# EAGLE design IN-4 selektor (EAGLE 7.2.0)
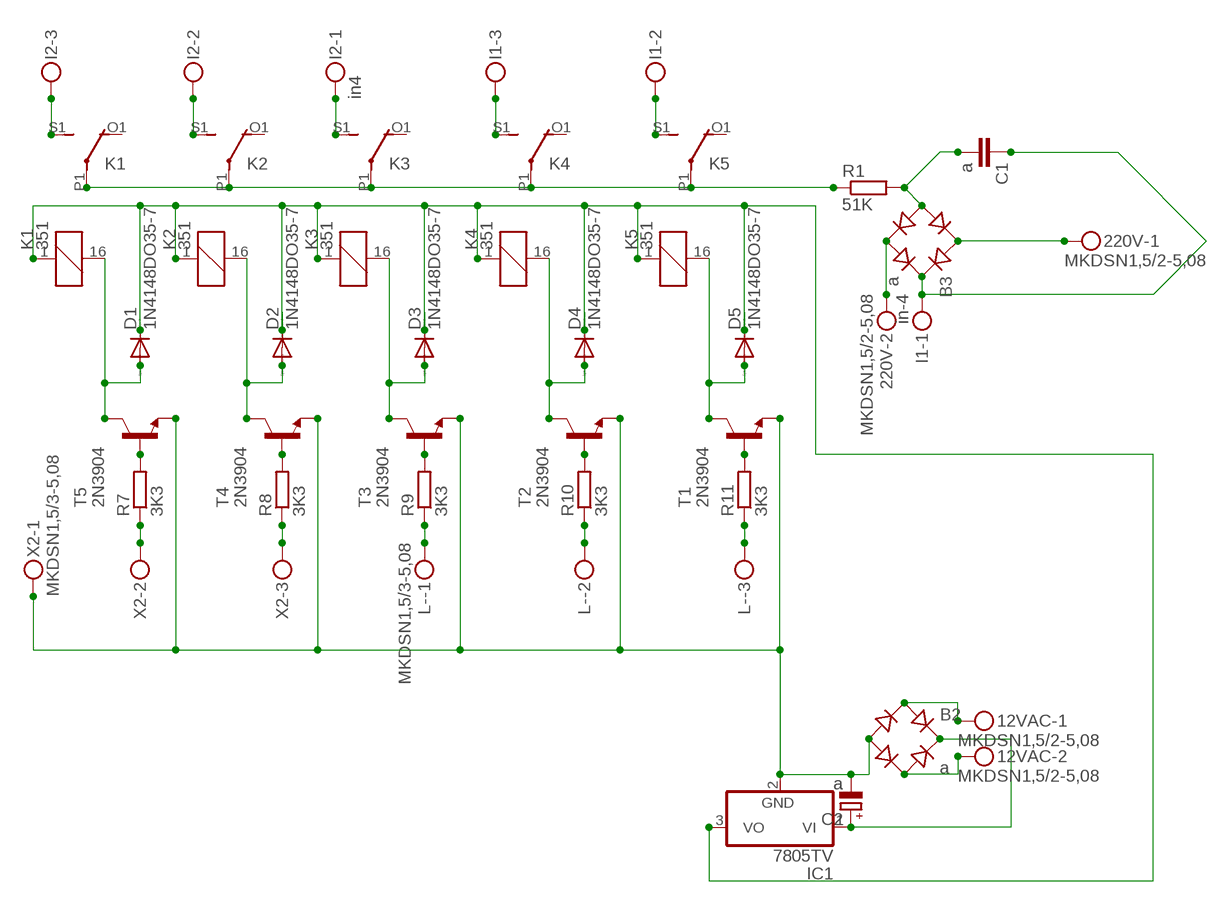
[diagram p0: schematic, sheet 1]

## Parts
12VAC  MKDSN1,5/2-5,08  [MKDSN1,5/2-5,08]
220V  MKDSN1,5/2-5,08  [MKDSN1,5/2-5,08]
B2  a  RB1A  [RB1A]
B3  a  RB1A  [RB1A]
C1  a  C-EU050-030X075  [C050-030X075]
C2  a  CPOL-EUE7.5-16  [E7,5-16]
D1  1N4148DO35-7  [DO35-7]
D2  1N4148DO35-7  [DO35-7]
D3  1N4148DO35-7  [DO35-7]
D4  1N4148DO35-7  [DO35-7]
D5  1N4148DO35-7  [DO35-7]
I1  in-4  MKDSN1,5/3-5,08  [MKDSN1,5/3-5,08]
I2  in4  MKDSN1,5/3-5,08  [MKDSN1,5/3-5,08]
IC1  7805TV  [TO220V]
K1  351  [351]
K2  351  [351]
K3  351  [351]
K4  351  [351]
K5  351  [351]
L-  MKDSN1,5/3-5,08  [MKDSN1,5/3-5,08]
R1  51K  R-EU_0207/10  [0207/10]
R7  3K3  R-EU_0204/5  [0204/5]
R8  3K3  R-EU_0204/5  [0204/5]
R9  3K3  R-EU_0204/5  [0204/5]
R10  3K3  R-EU_0204/5  [0204/5]
R11  3K3  R-EU_0204/5  [0204/5]
T1  2N3904  [TO92]
T2  2N3904  [TO92]
T3  2N3904  [TO92]
T4  2N3904  [TO92]
T5  2N3904  [TO92]
X2  MKDSN1,5/3-5,08  [MKDSN1,5/3-5,08]

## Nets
N$2: R8.2 T4.2(B)
N$3: R7.2 T5.2(B)
N$4: R9.2 T3.2(B)
N$5: R10.2 T2.2(B)
N$6: R11.2 T1.2(B)
N$7: 220V.1 B3.AC1
N$8: B3.+ C1.1 I1.1
N$9: K1.P1(2:P) K2.P1(2:P) K3.P1(2:P) K4.P1(2:P) K5.P1(2:P) R1.1
N$10: I2.3 K1.S1(2:S)
N$11: I2.2 K2.S1(2:S)
N$12: I2.1 K3.S1(2:S)
N$13: I1.3 K4.S1(2:S)
N$14: I1.2 K5.S1(2:S)
N$15: 220V.2 B3.AC2
N$16: R7.1 X2.2
N$17: B3.- C1.2 R1.2
N$19: B2.- C2.- IC1.2(GND) T1.3(E) T2.3(E) T3.3(E) T4.3(E) T5.3(E) X2.1
N$20: D1.A K1.16 T5.1(C)
N$22: R8.1 X2.3
N$23: L-.1 R9.1
N$25: D2.A K2.16 T4.1(C)
N$27: 12VAC.1 B2.AC1
N$28: 12VAC.2 B2.AC2
N$29: B2.+ C2.+ IC1.1(VI)
N$30: L-.2 R10.1
N$31: L-.3 R11.1
N$32: D3.A K3.16 T3.1(C)
N$34: D4.A K4.16 T2.1(C)
N$36: D5.A K5.16 T1.1(C)
N$37: D1.C D2.C D3.C D4.C D5.C IC1.3(VO) K1.1 K2.1 K3.1 K4.1 K5.1
Unconnected: K1.O1(2:O) K1.O2(3:O) K1.P2(3:P) K1.S2(3:S) K2.O1(2:O) K2.O2(3:O) K2.P2(3:P) K2.S2(3:S) K3.O1(2:O) K3.O2(3:O) K3.P2(3:P) K3.S2(3:S) K4.O1(2:O) K4.O2(3:O) K4.P2(3:P) K4.S2(3:S) K5.O1(2:O) K5.O2(3:O) K5.P2(3:P) K5.S2(3:S)

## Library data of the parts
12VAC 220V = con-phoenix-508:MKDSN1,5/2-5,08: MKDSN 1,5/ 2-5,08 Printklemme
B2 B3 = rectifier:RB1A: RECTIFIER 1 A
C1 = rcl:C-EU: CAPACITOR, European symbol
C2 = resistor:CPOL-EU: POLARIZED CAPACITOR, European symbol
D1-D5 = diode:1N4148: DIODE
I1 I2 L- X2 = con-phoenix-508:MKDSN1,5/3-5,08: MKDSN 1,5/ 3-5,08 Printklemme Nennstrom: 13,5 A Nennspannung: 250 V Rastermaß: 5,08 mm Polzahl: 3 Anschlussart: Schraubanschluss Montage: Löten Anschlussrichtung Leiter/Platine: 0 ° Artikelnummer: 1729131 Source: http://eshop.phoenixcontact.com .. 1729131.pdf
IC1 = linear:78*: Positive VOLTAGE REGULATOR Source: http://cache.national.com/ds/LM/LM78L05.pdf http://www.fairchildsemi.com/ds/LM/LM7805.pdf
K1-K5 = relay:351: RELAY 2 x switch, Omron; OC_FARNELL: unknown; OC_NEWARK: unknown
R1 R7-R11 = rcl:R-EU_: RESISTOR, European symbol
T1-T5 = transistor-neu-to92:2N3904: NPN TRANSISTOR

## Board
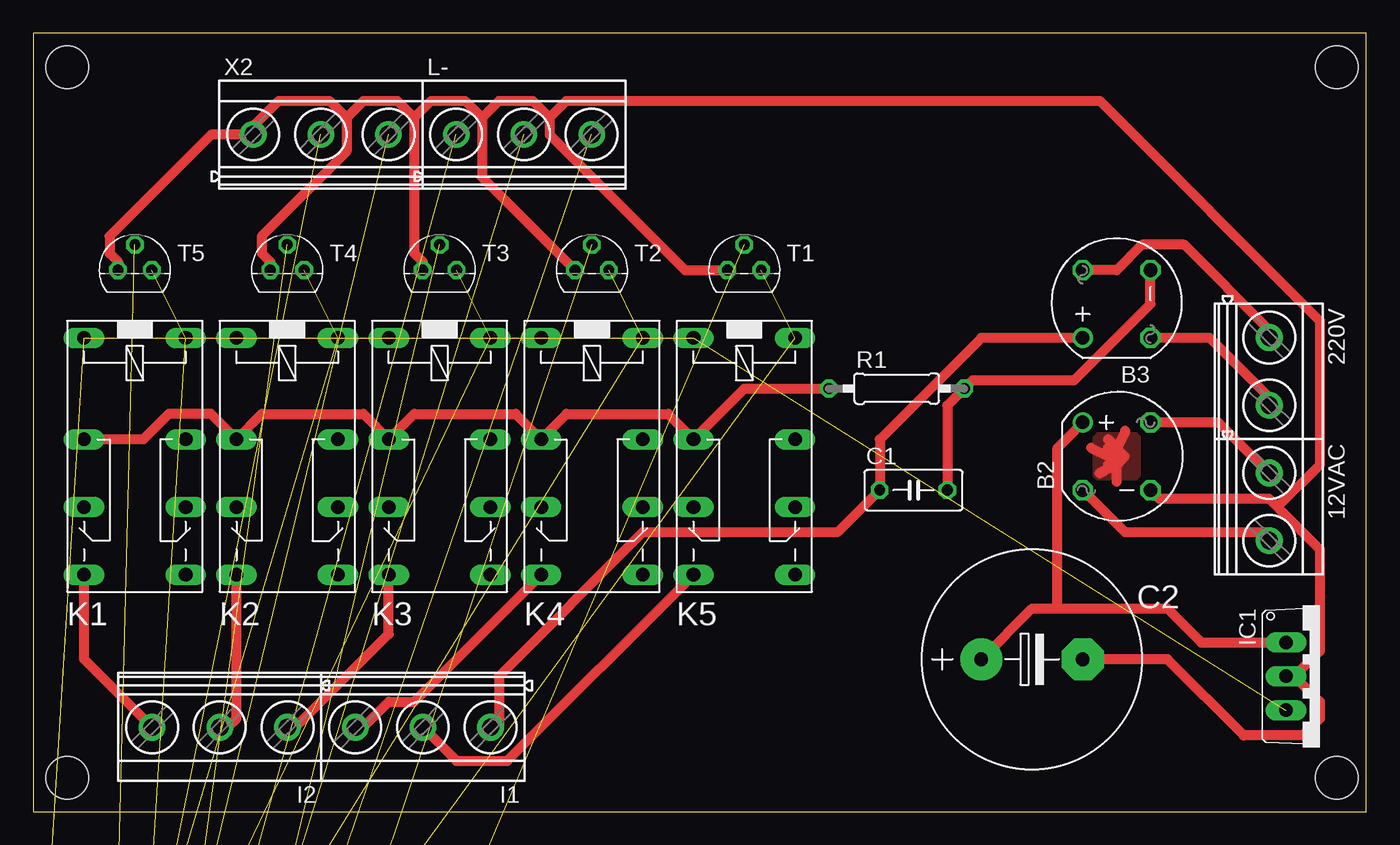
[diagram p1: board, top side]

Size 100 x 58.41 mm. Coordinates in mm from the lower left corner, seen from the top.
Outline: 0,0 100,0 100,58.41 0,58.41 0,0
Copper layers (1*16): Top 0.035mm / dielectric 1.5mm / Bottom 0.035mm
Design rules "default *": minimum track width 30mil, minimum drill 24mil, track to track 20mil, track to pad 20mil, pad to pad 20mil, via to via 20mil, smd to smd 20mil, copper to edge 50mil, drill to drill 20mil, minimum pad ring 10mil, minimum via ring 8mil, stop-mask expansion 4mil, vias tented up to drill 0mil, thermal gap 10mil
Holes 3.2 mm at 2.54,2.54 97.79,2.54 97.79,55.88 2.54,55.88

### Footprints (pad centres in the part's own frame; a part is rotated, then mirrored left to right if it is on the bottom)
MKDSN1,5/2-5,08 = drill 1.3 pad 2: 1 -2.561,0.025; 2 2.519,0.025
RB1A = drill 1.016: + -2.54,2.54 | drill 1.016 octagon: - 2.54,-2.54; AC1 2.54,2.54; AC2 -2.54,-2.54
C050-030X075 = drill 0.813 octagon: 1 -2.54,0; 2 2.54,0
E7,5-16 = drill 1.016 pad 3.15: + -3.81,0 | drill 1.016 pad 3.15 octagon: - 3.81,0
DO35-7 = drill 0.813 long: A 3.81,0; C -3.81,0
MKDSN1,5/3-5,08 = drill 1.3 pad 2: 1 -7.641,0.025; 2 -2.561,0.025; 3 2.519,0.025
TO220V = drill 1.016 long: 1 -2.54,-2.54; 2 0,-2.54; 3 2.54,-2.54
351 = drill 1.016 long: 1 -3.81,-3.81; 16 -3.81,3.81; O1 8.89,-3.81; O2 8.89,3.81; P1 3.81,-3.81; P2 3.81,3.81; S1 13.97,-3.81; S2 13.97,3.81
0207/10 = drill 0.813 octagon: 1 -5.08,0; 2 5.08,0
0204/5 = drill 0.813 octagon: 1 -2.54,0; 2 2.54,0
TO92 = drill 0.813 octagon: 1 1.27,0; 2 0,1.905; 3 -1.27,0

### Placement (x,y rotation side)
12VAC  92.71,22.86 270 top
220V  92.71,33.02 270 top
B2  81.28,26.67 0 top
B3  81.28,38.1 90 top
C1  66.04,24.13 0 top
C2  74.93,11.43 0 top
D1  not placed on the board
D2  not placed on the board
D3  not placed on the board
D4  not placed on the board
D5  not placed on the board
I1  26.67,6.35 180 top
I2  11.43,6.35 180 top
IC1  96.52,10.16 270 top
K1  7.62,31.75 270 top
K2  19.05,31.75 270 top
K3  30.48,31.75 270 top
K4  41.91,31.75 270 top
K5  53.34,31.75 270 top
L-  39.37,50.8 0 top
R1  64.77,31.75 0 top
R7  not placed on the board
R8  not placed on the board
R9  not placed on the board
R10  not placed on the board
R11  not placed on the board
T1  53.34,40.64 0 top
T2  41.91,40.64 0 top
T3  30.48,40.64 0 top
T4  19.05,40.64 0 top
T5  7.62,40.64 0 top
X2  24.13,50.8 0 top

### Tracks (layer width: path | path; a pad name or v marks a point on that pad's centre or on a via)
N$1
  Top 0.762: 80.64,27.3 81.28,27.26 | 81.28,24.77 81.28,26.03 | 81.28,26.03 81.28,26.08 80.01,25.4 | 80.64,27.94 81.28,27.26 | 81.28,27.3 81.28,27.26 | 80.64,26.03 81.58,26.96 | 79.38,27.3 80.69,26.67 | 81.28,26.03 81.87,26.67 | 80.64,26.67 81.28,27.26 | 81.92,28.58 81.28,27.26
  pour Top: 0,58.42 100.33,58.42 100.33,0 0,0
N$2  (1 unrouted)
N$3  (1 unrouted)
N$4  (1 unrouted)
N$5  (1 unrouted)
N$6  (1 unrouted)
N$7
  Top 0.762: B3.AC1 81.28,40.64 83.19,42.55 86.36,42.55 92.71,36.2 220V.1
N$8
  Top 0.762: B3.+ 71.12,35.56 63.5,27.94 C1.1 60.33,20.95 45.72,20.95 34.92,10.16 34.92,6.35 I1.1
N$9
  Top 0.762: R1.1 53.34,31.75 K5.P1 47.62,29.84 40.01,29.84 K4.P1 36.2,29.84 28.57,29.84 K3.P1 24.77,29.84 17.14,29.84 K2.P1 13.34,29.84 10.16,29.84 8.26,27.94 K1.P1
N$10
  Top 0.762: K1.S1 3.81,11.43 8.89,6.35 I2.3
N$11
  Top 0.762: K2.S1 15.24,6.98 14.61,6.35 I2.2
N$12
  Top 0.762: K3.S1 26.67,13.34 19.68,6.35 I2.1
N$13
  Top 0.762: K4.S1 28.57,8.25 26.67,8.25 24.77,6.35 I1.3
N$14
  Top 0.762: K5.S1 35.56,3.81 31.75,3.81 29.84,5.71 I1.2
N$15
  Top 0.762: B3.AC2 88.27,35.56 92.71,31.12 220V.2
N$16  (1 unrouted)
N$17
  Top 0.762: C1.2 68.58,30.48 R1.2 70.48,32.38 78.11,32.38 83.82,38.1 B3.-
N$19
  Top 0.762: 94.61,10.16 96.52,12.06 96.52,19.69 93.34,22.86 | 93.34,22.86 92.71,23.49 84.45,23.49 B2.- | C2.- 85.09,11.43 90.81,5.71 95.25,5.71 96.52,6.98 96.52,8.25 94.61,10.16 | 94.61,10.16 IC1.2 | T5.3 6.35,41.27 5.71,41.91 5.71,43.18 13.34,50.8 15.88,50.8 X2.1 16.51,51.43 18.41,53.34 22.23,53.34 23.5,52.07 | T4.3 17.78,41.27 17.14,41.91 17.14,43.18 23.5,49.53 23.5,52.07 | T3.3 29.21,41.27 28.57,41.91 28.57,52.07 | 28.57,52.07 27.3,53.34 24.77,53.34 23.5,52.07 | T2.3 33.66,47.62 33.66,52.07 | 33.66,52.07 32.38,53.34 29.84,53.34 28.57,52.07 | T1.3 48.9,40.64 38.73,50.8 38.73,52.07 | 38.73,52.07 37.47,53.34 34.92,53.34 33.66,52.07 | 93.34,22.86 96.52,26.03 96.52,36.83 80.01,53.34 40.01,53.34 38.73,52.07
N$20  (2 unrouted)
N$22  (1 unrouted)
N$23  (1 unrouted)
N$25  (2 unrouted)
N$27
  Top 0.762: B2.AC1 88.9,29.21 92.71,25.4 12VAC.1
N$28
  Top 0.762: B2.AC2 81.92,20.95 92.71,20.95 12VAC.2
N$29
  Top 0.762: IC1.1 87.63,12.7 85.09,15.24 76.83,15.24 | 76.83,15.24 74.93,15.24 C2.+ | B2.+ 76.83,27.3 76.83,15.24
N$30  (1 unrouted)
N$31  (1 unrouted)
N$32  (2 unrouted)
N$34  (2 unrouted)
N$36  (2 unrouted)
N$37  (10 unrouted)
